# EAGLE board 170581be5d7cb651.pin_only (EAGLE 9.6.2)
REVISION: A

Size 25.4 x 25.4 mm. Coordinates in mm from the lower left corner, seen from the top.
Outline: 0,0 0,25.4 25.4,25.4 25.4,0 0,0
Copper layers (1*16): Top 0.035mm / dielectric 1.5mm / Bottom 0.035mm
Design rules "SparkFun-2-Layer-Minimum-JLCPCB": minimum track width 5mil, minimum drill 0.3mm, track to track 5mil, track to pad 5mil, pad to pad 5mil, via to via 5mil, smd to smd 5mil, copper to edge 7mil, drill to drill 7mil, minimum pad ring 5mil, minimum via ring 5mil, stop-mask expansion 2.5mil, vias tented up to drill 25mil, thermal gap 10mil
Net classes: 1 power: width 0.203 mm

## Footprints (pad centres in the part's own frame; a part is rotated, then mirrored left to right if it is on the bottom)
0603 = smd 1.1 x 1: 1 -0.85,0; 2 0.85,0
LED-0603 = smd 1 x 1: A -0.877,0; C 0.877,0
SMT-JUMPER_3_2-NC_TRACE_SILK = smd 0.66 x 1.27: 1 -1.041,0; 2 0,0; 3 1.041,0
SMT-JUMPER_2_NC_TRACE_SILK = smd 0.66 x 1.27: 1 -0.521,0; 2 0.521,0
JST04_1MM_RA = smd 0.6 x 1.35: 1 -1.5,0; 2 -0.5,0; 3 0.5,0; 4 1.5,0 | smd 1.2 x 2: NC1 2.8,-3.675; NC2 -2.8,-3.675
1X04_NO_SILK = drill 1.016 pad 1.88: 1 0,0; 2 2.54,0; 3 5.08,0; 4 7.62,0
1X01_NO_SILK = drill 1.016 pad 1.88: 1 0,0
FIDUCIAL-1X2 = smd 1 x 1: 1 0,0
STAND-OFF = hole 3.302: 0,0
SOT23-3 = smd 0.8 x 0.9: 1 -0.95,-1; 2 0.95,-1; 3 0,1.1
SOT353 = smd 0.42 x 0.7: 1 -0.65,-0.95; 2 0,-0.95; 3 0.65,-0.95; 4 0.65,0.95; 5 -0.65,0.95
MSOP8 = smd 1.1 x 0.4: 1 -2.25,0.975; 2 -2.25,0.325; 3 -2.25,-0.325; 4 -2.25,-0.975; 5 2.25,-0.975; 6 2.25,-0.325; 7 2.25,0.325; 8 2.25,0.975
VSSOP_8PIN = smd 0.8 x 0.3: P1 -1.55,0.75; P2 -1.55,0.25; P3 -1.55,-0.25; P4 -1.55,-0.75; P5 1.55,-0.75; P6 1.55,-0.25; P7 1.55,0.25; P8 1.55,0.75

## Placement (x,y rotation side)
C1  0.1uF  [0603]  7.62,10.79 270 top
C2  10uF  [0603]  9.14,16.89 90 top
C3  0.1uF  [0603]  18.29,9.91 270 top
D1  RED  [LED-0603]  2.54,17.14 0 top
D2  GREEN  [LED-0603]  22.86,8.26 180 top
FRAME1  FRAME-LETTER  [CREATIVE_COMMONS]  not placed on the board
I2C_IN  JUMPER-SMT_3_2-NC_TRACE_SILK  [SMT-JUMPER_3_2-NC_TRACE_SILK]  3.17,4.19 90 bottom
I2C_OUT  JUMPER-SMT_3_2-NC_TRACE_SILK  [SMT-JUMPER_3_2-NC_TRACE_SILK]  21.97,17.78 270 bottom
IN_LED  IN_LED  [SMT-JUMPER_2_NC_TRACE_SILK]  5.08,17.78 180 bottom
J1  Qwiic Right Angle  [JST04_1MM_RA]  5.08,12.7 270 top
J2  PTH  [1X04_NO_SILK]  15.24,1.27 0 bottom
J3  Qwiic Right Angle  [JST04_1MM_RA]  20.32,12.7 90 top
J4  PTH  [1X04_NO_SILK]  10.16,24.13 0 top
J5  [1X01_NO_SILK]  17.78,1.27 0 top
J6  [1X01_NO_SILK]  7.62,24.13 0 top
JP1  FIDUCIAL1X2  [FIDUCIAL-1X2]  0.76,24.64 0 bottom
JP2  FIDUCIAL1X2  [FIDUCIAL-1X2]  24.51,0.89 0 top
JP3  STAND-OFF  [STAND-OFF]  2.54,22.86 0 top
JP4  STAND-OFF  [STAND-OFF]  22.86,22.86 0 top
JP5  FIDUCIAL1X2  [FIDUCIAL-1X2]  24.51,0.89 0 bottom
JP6  FIDUCIAL1X2  [FIDUCIAL-1X2]  0.76,24.64 0 top
LOGO1  OSHW-LOGOMINI  [OSHW-LOGO-MINI]  22.23,3.81 0 bottom
LOGO2  SFE_LOGO_FLAME.1_INCH  [SFE_LOGO_FLAME_.1]  22.23,3.68 0 top
LOGO3  SFE_LOGO_NAME_FLAME.1_INCH  [SFE_LOGO_NAME_FLAME_.1]  12.7,15.24 0 bottom
OUT_LED  OUT_LED  [SMT-JUMPER_2_NC_TRACE_SILK]  20.32,7.62 0 bottom
Q1  20V/4.2A/52mΩ/1.4W  [SOT23-3]  11.94,17.14 180 top
R1  1k  [0603]  2.54,19.05 0 top
R2  470  [0603]  22.86,6.35 180 top
R3  2.2k  [0603]  3.17,6.35 180 top
R4  2.2k  [0603]  3.17,3.68 180 top
R5  1k  [0603]  15.75,17.4 90 top
R6  2.2k  [0603]  17.78,17.4 270 top
R7  2.2k  [0603]  21.97,19.05 0 top
R8  200k  [0603]  10.79,10.16 180 top
U1  74HC1G04  [SOT353]  14.99,8.89 90 top
U2  PCA9536  [MSOP8]  12.7,12.7 180 top
U3  [VSSOP_8PIN]  10.79,8 0 top
U$1  [IN0]  1.52,3.94 90 bottom
U$3  [GND1]  10.16,23.75 270 top
U$4  [3#3V0]  12.7,1.65 90 bottom
U$5  [SDA8]  15.24,23.75 270 top
U$6  [SCL9]  17.78,23.75 270 top
U$7  [3#3V0]  12.7,23.75 270 bottom
U$8  [GND1]  15.24,1.65 90 bottom
U$9  [SCL9]  7.62,1.65 90 bottom
U$10  [I_SUPER2_C-()-03]  1.52,1.78 90 bottom
U$11  [SDA8]  10.16,1.65 90 bottom
U$12  [3#3V0]  12.7,23.75 270 top
U$13  [GND1]  15.24,1.65 90 top
U$14  [OUT0]  23.62,18.16 270 bottom
U$15  [SDA8]  10.16,1.65 90 top
U$16  [GPIO10]  17.78,1.65 90 bottom
U$17  [SCL9]  7.62,1.65 90 top
U$18  [I_SUPER2_C-()-03]  23.62,20.32 270 bottom
U$19  [QWIIC0]  16,13.46 0 bottom
U$20  [GPIO20]  7.62,23.88 270 bottom
U$22  [GND1]  10.16,23.75 270 bottom
U$23  [3#3V0]  12.7,1.65 90 top
U$24  [GPIO10]  17.78,1.65 90 top
U$25  [GPIO20]  7.62,23.88 270 top
U$26  [SCL9]  17.78,23.75 270 bottom
U$27  [SDA8]  15.24,23.75 270 bottom
U$28  [IN0]  0.64,8.26 0 top
U$29  [LED_IN0]  3.3,15.49 90 bottom
U$30  [LED_OUT0]  23.37,9.27 0 bottom
U$31  [OUT0]  19.56,17.14 0 top
U$32  [POWER0]  16.38,11.56 0 bottom
U$34  [SWITCH0]  16.51,9.53 0 bottom

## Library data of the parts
C1 C3 = SparkFun-Capacitors; PROD_ID: CAP-00810
C2 = SparkFun-Capacitors; PROD_ID: CAP-11015
D1 = SparkFun-LED; PROD_ID: DIO-00819
D2 = SparkFun-LED; PROD_ID: DIO-00821
FRAME1 JP1 JP2 JP5 JP6 LOGO1-LOGO3 = SparkFun-Aesthetics
I2C_IN I2C_OUT IN_LED OUT_LED = SparkFun-Jumpers
J1 J3 = SparkFun-Connectors; PROD_ID: CONN-13694
J2 J4-J6 = SparkFun-Connectors
JP3 JP4 = SparkFun-Hardware
Q1 = SparkFun-DiscreteSemi; PROD_ID: TRANS-14388
R1 R5 = SparkFun-Resistors; PROD_ID: RES-07856
R2 = SparkFun-Resistors; PROD_ID: RES-07869
R3 R4 R6 R7 = SparkFun-Resistors; PROD_ID: RES-08272
R8 = SparkFun-Resistors; PROD_ID: RES-09385
U1 = SparkFun-IC-Logic; PROD_ID: COMP-08268
U2 = SparkFun-IC-Conversion; PROD_ID: IC-15034
U3 = SparkFun-IC-Comms; PROD_ID: IC-14450
U$1 = IN__3
U$3 U$5 U$6 U$8 U$9 U$11 U$13 U$15 U$17 U$22 U$26 U$27 = Labels-0_04
U$4 U$23 = 3.3V_Pointer
U$7 U$12 = 3.3V_Flagtail
U$10 U$18 = Labels
U$14 = OUT__3
U$16 U$24 = GPIO1
U$19 = Qwiic
U$20 U$25 = GPIO2
U$28 = IN
U$29 = LED_IN
U$30 = LED_OUT
U$31 = OUT
U$32 = Power
U$34 = switch

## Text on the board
Bottom: v10
Document: Measurements in inches.
tDocu: Paul Clark

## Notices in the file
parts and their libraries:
SparkFun-Resistors: Licensing: Creative Commons ShareAlike 4.0 International - https://creativecommons.org/licenses/by-sa/4.0
SparkFun-Aesthetics: Released under the Creative Commons Attribution Share-Alike 4.0 License
SparkFun-Aesthetics: https://creativecommons.org/licenses/by-sa/4.0
